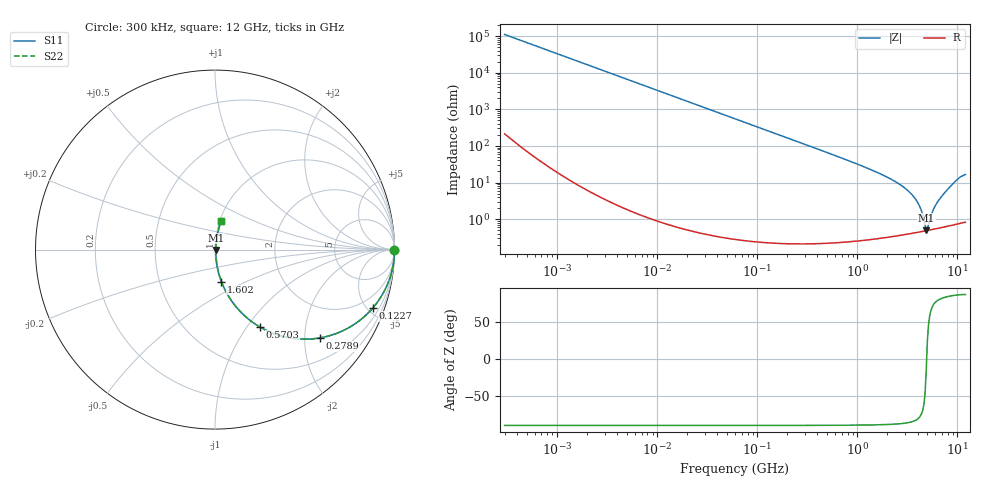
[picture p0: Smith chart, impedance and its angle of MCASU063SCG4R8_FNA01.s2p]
! MCASU063SCG4R8_FNA01  S-PARAMETER MODEL  ( General Type )
! Model Generated by TAIYO YUDEN Corporation (http://www.ty-top.com)
! Version 2.0
! TAIYO YUDEN Control No. 141201
! Copyright(c) 2013 TAIYO YUDEN CO.,LTD. All Rights Reserved.
! Product Description (link to TY-COMPAS)
! https://ds.yuden.co.jp/TYCOMPAS/or/detail?pn=MCASU063SCG4R8CFNA01&u=M
! Products Name : Multilayer Ceramic Capacitors
! Characteristics :
!  Capacitance : 4.8 pF , Rated Voltage : 50V , TCC : CG / C0G
!  Case Size : 0.6 x 0.3 / 0.024 x 0.012 [mm/inch] , Thickness : 0.3 / 0.012 [mm/inch]
!  (Conditions: Temperature = 25 degC , DC Bias Current/Voltage = 0A / 0V)
! External Node Assignments :
!  1  o---| |---o  2
! GND o---------o GND
! Frequency Range : 0.3MHz  -  12000MHz  [ 401 STEP ]
# MHz S RI R 50
! Freq[MHz].  S11 Real  S11 Imag  S21 Real  S21 Imag  S12 Real  S12 Imag  S22 Real  S22 Imag
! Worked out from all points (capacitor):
!   401 points, 300 kHz to 12 GHz, reference 50 ohm
!   read as one part in series: C = 4.79 pF near 316.3 kHz
!   lowest |Z| = 501 mohm at 4.875 GHz (marker M1)
!   series resonance near 4.924 GHz, so ESL is about 220 pH
!   S11 on the Smith chart (normalised r, x): 300 kHz: open; 122.7 MHz: 1.00, -5.41; 278.9 MHz: 1.00, -2.37; 570.3 MHz: 1.00, -1.15; 1.602 GHz: 1.01, -0.37; 12 GHz: 1.02, +0.33
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0.3  1 -0.000904  2.56e-06 0.000904  2.56e-06 0.000904  1 -0.000904
1.769972  1 -0.00533  3.05e-05 0.00533  3.05e-05 0.00533  1 -0.00533
10.44266  0.999 -0.0314  0.000997 0.0314  0.000997 0.0314  0.999 -0.0314
60  0.9683 -0.175  0.0317 0.175  0.0317 0.175  0.9683 -0.175
122.6847  0.8795 -0.3252  0.1205 0.3252  0.1205 0.3252  0.8795 -0.3252
278.9009  0.5845 -0.4919  0.4155 0.4919  0.4155 0.4919  0.5845 -0.4919
353.9943  0.4654 -0.4977  0.5346 0.4977  0.5346 0.4977  0.4654 -0.4977
570.2811  0.2488 -0.4304  0.7512 0.4304  0.7512 0.4304  0.2488 -0.4304
918.7169  0.1101 -0.3096  0.8899 0.3096  0.8899 0.3096  0.1101 -0.3096
1602.47  0.0358 -0.1781  0.9642 0.1781  0.9642 0.1781  0.0358 -0.1781
2088.533  0.0198 -0.1274  0.9802 0.1274  0.9802 0.1274  0.0198 -0.1274
2870.14  0.00943 -0.0754  0.9906 0.0754  0.9906 0.0754  0.00943 -0.0754
3642.919  0.00581 -0.0409  0.9942 0.0409  0.9942 0.0409  0.00581 -0.0409
4158.869  0.00493 -0.0227  0.9951 0.0227  0.9951 0.0227  0.00493 -0.0227
4385.161  0.00478 -0.0156  0.9952 0.0156  0.9952 0.0156  0.00478 -0.0156
4747.894  0.00475 -0.00492  0.9952 0.00492  0.9952 0.00492  0.00475 -0.00492
4875.354  0.0048 -0.00134  0.9952 0.00134  0.9952 0.00134  0.0048 -0.00134
5140.631  0.00496 0.0051  0.995 -0.0051  0.995 -0.0051  0.00496 0.0051
5868.704  0.00569 0.0196  0.9943 -0.0196  0.9943 -0.0196  0.00569 0.0196
6879.757  0.00737 0.0394  0.9926 -0.0394  0.9926 -0.0394  0.00737 0.0394
9708.23  0.0195 0.1103  0.9805 -0.1103  0.9805 -0.1103  0.0195 0.1103
12000  0.0341 0.1581  0.9659 -0.1581  0.9659 -0.1581  0.0341 0.1581
